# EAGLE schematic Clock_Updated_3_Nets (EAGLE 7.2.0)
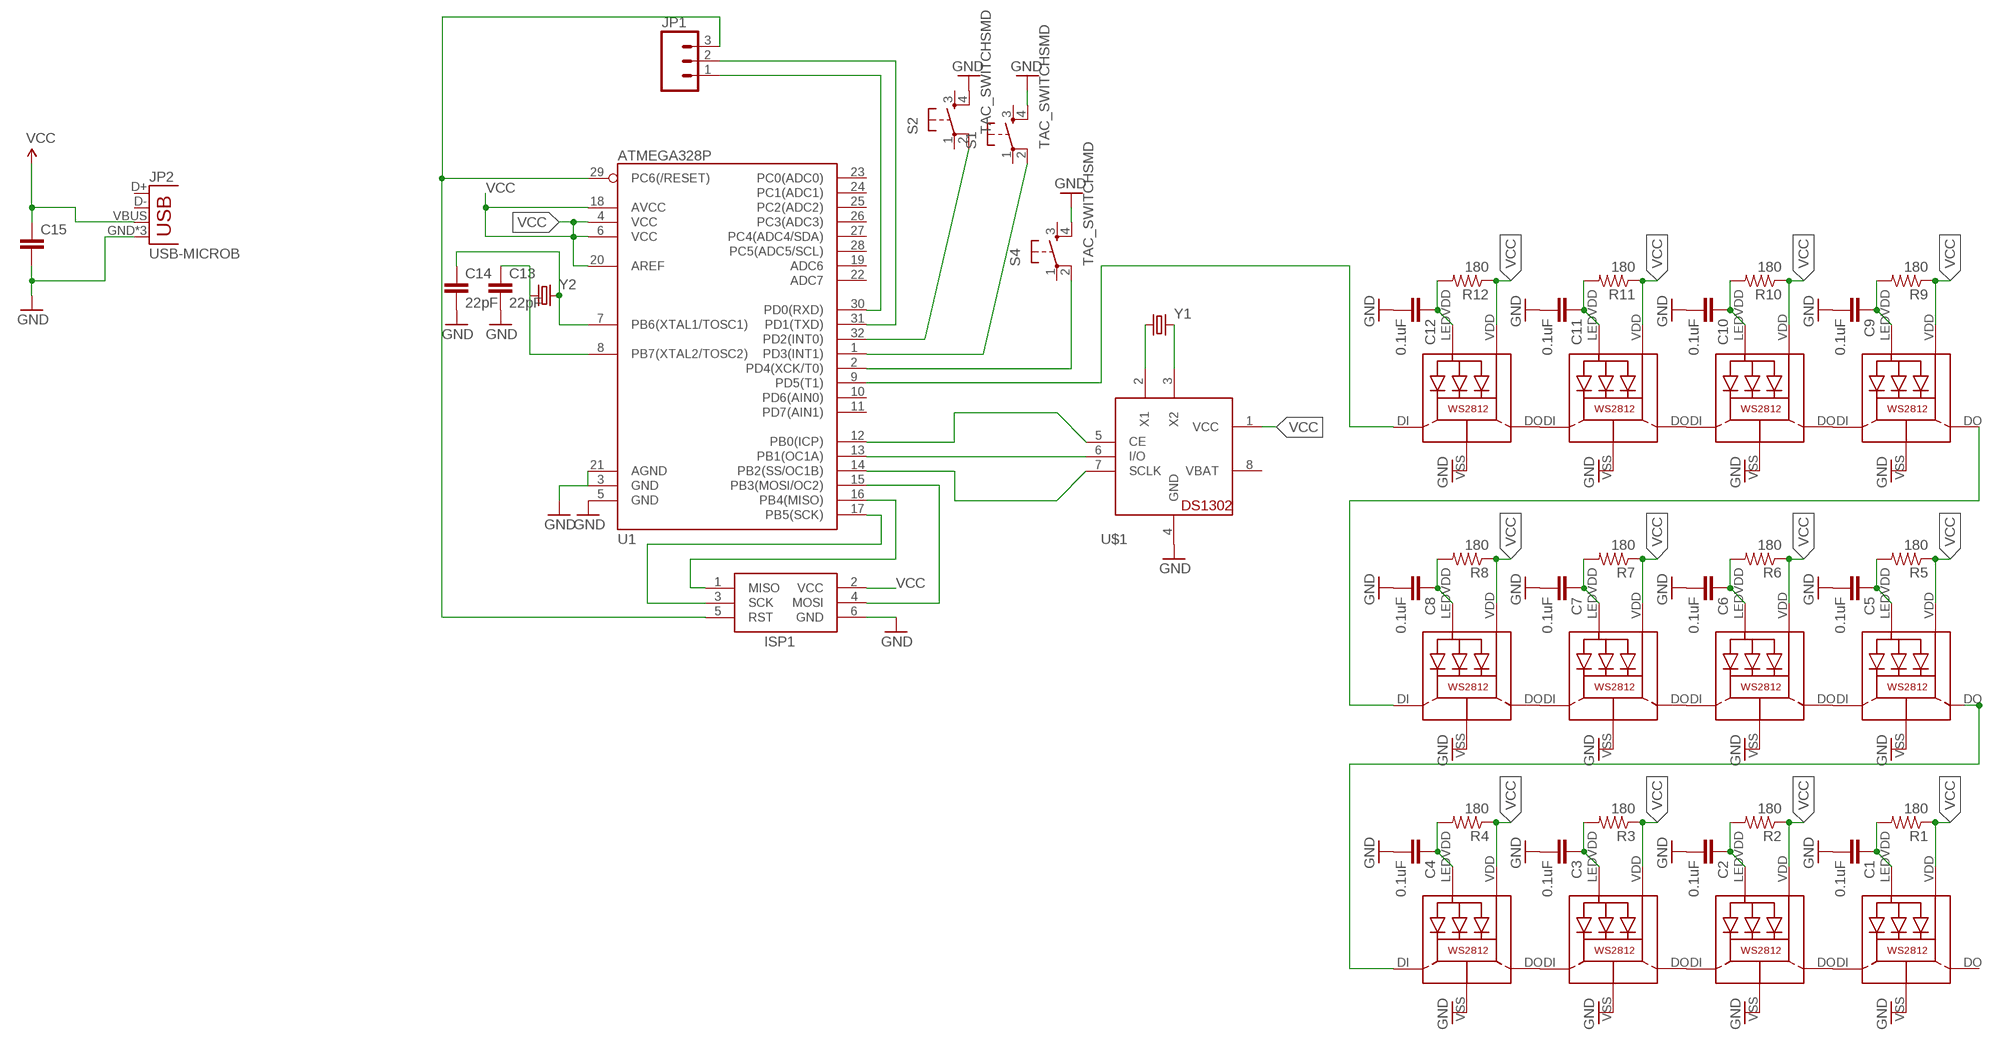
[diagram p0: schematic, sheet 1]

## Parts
C1  0.1uF  0.1UF-25V(+80/-20%)(0603)  [0603-CAP]
C2  0.1uF  0.1UF-25V(+80/-20%)(0603)  [0603-CAP]
C3  0.1uF  0.1UF-25V(+80/-20%)(0603)  [0603-CAP]
C4  0.1uF  0.1UF-25V(+80/-20%)(0603)  [0603-CAP]
C5  0.1uF  0.1UF-25V(+80/-20%)(0603)  [0603-CAP]
C6  0.1uF  0.1UF-25V(+80/-20%)(0603)  [0603-CAP]
C7  0.1uF  0.1UF-25V(+80/-20%)(0603)  [0603-CAP]
C8  0.1uF  0.1UF-25V(+80/-20%)(0603)  [0603-CAP]
C9  0.1uF  0.1UF-25V(+80/-20%)(0603)  [0603-CAP]
C10  0.1uF  0.1UF-25V(+80/-20%)(0603)  [0603-CAP]
C11  0.1uF  0.1UF-25V(+80/-20%)(0603)  [0603-CAP]
C12  0.1uF  0.1UF-25V(+80/-20%)(0603)  [0603-CAP]
C13  22pF  22PF-50V-5%(0603)  [0603-CAP]
C14  22pF  22PF-50V-5%(0603)  [0603-CAP]
C15  CAP1206  [1206]
ISP1  AVRISP-6  [AVRISP]
JP1  M03JST-PTH-VERT  [JST-3-PTH-VERT]
JP2  USB-MICROB  [USB-MICROB]
LED1  WS2812  [WS2812]
LED2  WS2812  [WS2812]
LED3  WS2812  [WS2812]
LED4  WS2812  [WS2812]
LED5  WS2812  [WS2812]
LED6  WS2812  [WS2812]
LED7  WS2812  [WS2812]
LED8  WS2812  [WS2812]
LED9  WS2812  [WS2812]
LED10  WS2812  [WS2812]
LED11  WS2812  [WS2812]
LED12  WS2812  [WS2812]
R1  180  180OHM1/10W1%(0603)  [0603-RES]
R2  180  180OHM1/10W1%(0603)  [0603-RES]
R3  180  180OHM1/10W1%(0603)  [0603-RES]
R4  180  180OHM1/10W1%(0603)  [0603-RES]
R5  180  180OHM1/10W1%(0603)  [0603-RES]
R6  180  180OHM1/10W1%(0603)  [0603-RES]
R7  180  180OHM1/10W1%(0603)  [0603-RES]
R8  180  180OHM1/10W1%(0603)  [0603-RES]
R9  180  180OHM1/10W1%(0603)  [0603-RES]
R10  180  180OHM1/10W1%(0603)  [0603-RES]
R11  180  180OHM1/10W1%(0603)  [0603-RES]
R12  180  180OHM1/10W1%(0603)  [0603-RES]
S1  TAC_SWITCHSMD  [TACTILE-SWITCH-SMD]
S2  TAC_SWITCHSMD  [TACTILE-SWITCH-SMD]
S4  TAC_SWITCHSMD  [TACTILE-SWITCH-SMD]
U1  ATMEGA328P  ATMEGA328_SMT  [TQFP32-08]
U$1  DS1302  [DIL08-ROUND]
Y1  CRYSTALTC38H  [TC38H]
Y2  CRYSTALSMD  [HC49UP]

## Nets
GND: C1.2 C2.2 C3.2 C4.2 C5.2 C6.2 C7.2 C8.2 C9.2 C10.2 C11.2 C12.2 C13.2 C14.2 C15.2 ISP1.6(GND) JP2.GND JP2.MT1(GND) JP2.MT2(GND) LED1.VSS(GND) LED2.VSS(GND) LED3.VSS(GND) LED4.VSS(GND) LED5.VSS(GND) LED6.VSS(GND) LED7.VSS(GND) LED8.VSS(GND) LED9.VSS(GND) LED10.VSS(GND) LED11.VSS(GND) LED12.VSS(GND) S1.4 S2.4 S4.4 U1.3(GND) U1.5(GND) U1.21(AGND) U$1.4(GND)
N$1: ISP1.4(MOSI) U1.15(PB3(MOSI/OC2))
N$2: ISP1.1(MISO) U1.16(PB4(MISO))
N$3: JP1.1 U1.30(PD0(RXD))
N$4: S2.2 U1.32(PD2(INT0))
N$5: U$1.3(X2) Y1.2
N$6: U$1.2(X1) Y1.1
N$7: C1.1 LED1.LEDVDD R1.2
N$8: C2.1 LED2.LEDVDD R2.2
N$9: LED1.DI LED2.DO
N$10: C3.1 LED3.LEDVDD R3.2
N$11: C4.1 LED4.LEDVDD R4.2
N$12: LED3.DI LED4.DO
N$13: C5.1 LED5.LEDVDD R5.2
N$14: C6.1 LED6.LEDVDD R6.2
N$15: LED5.DI LED6.DO
N$16: C7.1 LED7.LEDVDD R7.2
N$17: C8.1 LED8.LEDVDD R8.2
N$18: LED7.DI LED8.DO
N$19: C9.1 LED9.LEDVDD R9.2
N$20: C10.1 LED10.LEDVDD R10.2
N$21: LED9.DI LED10.DO
N$22: C11.1 LED11.LEDVDD R11.2
N$23: C12.1 LED12.LEDVDD R12.2
N$24: LED11.DI LED12.DO
N$25: LED4.DI LED5.DO
N$26: LED8.DI LED9.DO
N$27: JP1.2 U1.31(PD1(TXD))
N$30: S1.2 U1.1(PD3(INT1))
N$31: U1.13(PB1(OC1A)) U$1.6(I/O)
N$32: U1.12(PB0(ICP)) U$1.5(CE)
N$33: U1.14(PB2(SS/OC1B)) U$1.7(SCLK)
N$34: ISP1.3(SCK) U1.17(PB5(SCK))
N$36: ISP1.5(RST) JP1.3 U1.29(PC6(/RESET))
N$37: S4.2 U1.2(PD4(XCK/T0))
N$38: C13.1 U1.8(PB7(XTAL2/TOSC2)) Y2.1
N$40: LED2.DI LED3.DO
N$41: LED6.DI LED7.DO
N$42: LED10.DI LED11.DO
N$43: LED12.DI U1.9(PD5(T1))
N$44: C14.1 U1.7(PB6(XTAL1/TOSC1)) Y2.2
VCC: C15.1 ISP1.2(VCC) JP2.VBUS LED1.VDD LED2.VDD LED3.VDD LED4.VDD LED5.VDD LED6.VDD LED7.VDD LED8.VDD LED9.VDD LED10.VDD LED11.VDD LED12.VDD R1.1 R2.1 R3.1 R4.1 R5.1 R6.1 R7.1 R8.1 R9.1 R10.1 R11.1 R12.1 U1.4(VCC) U1.6(VCC) U1.18(AVCC) U1.20(AREF) U$1.1(VCC)
Unconnected: JP2.D+ JP2.D- LED1.DO S1.1 S1.3 S2.1 S2.3 S4.1 S4.3 U1.10(PD6(AIN0)) U1.11(PD7(AIN1)) U1.19(ADC6) U1.22(ADC7) U1.23(PC0(ADC0)) U1.24(PC1(ADC1)) U1.25(PC2(ADC2)) U1.26(PC3(ADC3)) U1.27(PC4(ADC4/SDA)) U1.28(PC5(ADC5/SCL))

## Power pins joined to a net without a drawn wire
VBAT: U$1.8(VBAT)

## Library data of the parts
C1-C12 = SparkFun-Capacitors:0.1UF-25V(+80/-20%)(0603): CAP-00810; PROD_ID: CAP-00810
C13 C14 = SparkFun-Capacitors:22PF-50V-5%(0603): CAP-07876; PROD_ID: CAP-07876
C15 = SparkFun-Passives:CAP: Capacitor
ISP1 = adafruit:AVRISP: AVR ISP HEADER Standard 6 pin header for AVR programming
JP1 = SparkFun-Connectors:M03: Header 3 Standard 3-pin 0.1" header. Use with straight break away headers (SKU : PRT-00116), right angle break away headers (PRT-00553), swiss pins (PRT-00743), machine pins (PRT-00117), and female headers (PRT-00115). Molex polarized connector foot print use with SKU : PRT-08232 with associated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
JP2 = SparkFun-Connectors:USB: USB Connectors USB-B-PTH is fully proven SKU : PRT-00139/CONN-08278 USB-miniB is fully proven SKU : PRT-00587 USB-A-PCB is untested. USB-A-H is throughly reviewed, but untested. Spark Fun Electronics SKU : PRT-00437 USB-B-SMT is throughly reviewed, but untested. Needs silkscreen touching up.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; PROD_ID: CONN-09505
LED1-LED12 = adafruit:WS2812
R1-R12 = SparkFun-Resistors:180OHM1/10W1%(0603): RES-08788; PROD_ID: RES-08788
S1 S2 S4 = SparkFun-Electromechanical:TAC_SWITCH: Momentary Switch Button commonly used for reset or general input. Spark Fun Electronics SKU : COM-00097 SMT- SWCH-08247; PROD_ID: SWCH-08247
U1 = SparkFun-DigitalIC:ATMEGA328_SMT: 32-Pin Atmega328 part Commonly used on Arduino compatible boards Available in QFP and QFN packages TQFP is IC-09069 QFN is non-stock; PROD_ID: IC-09069
U$1 = adafruit:DS1302: DS1302 - Real time clock with supercap trickle charger
Y1 Y2 = SparkFun-FreqCtrl:CRYSTAL: Various standard crystals. Proven footprints. Spark Fun Electronics SKU : COM-00534

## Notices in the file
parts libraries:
SparkFun-FreqCtrl: Licensing: Creative Commons ShareAlike 4.0 International - https://creativecommons.org/licenses/by-sa/4.0
